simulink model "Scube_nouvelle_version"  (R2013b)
settings: Solver=ode23t  StartTime=0.0  StopTime=100  RelTol=1e-3
libraries: fl_lib x14, nesl_utility x7

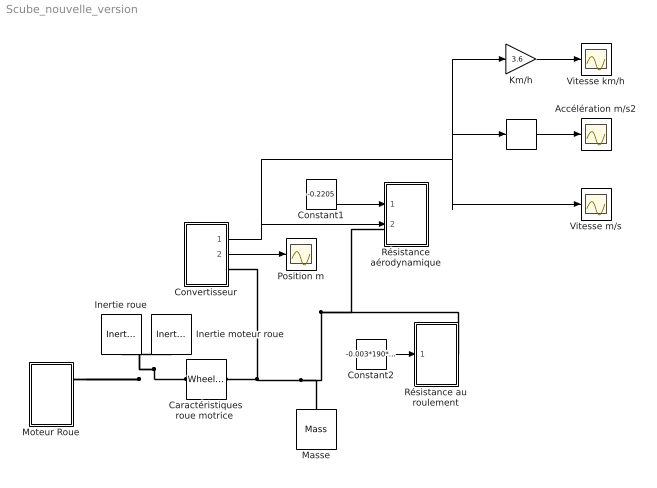
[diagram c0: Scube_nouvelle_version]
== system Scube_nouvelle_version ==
  " " : Derivative
  Accélération m/s2 : Scope
  "Caractéristiques roue motrice " : fl_lib/Mechanical/Mechanisms/Wheel and Axle  R=50 mm  or=1  orient=1  t_Log=off  f_Log=off  LocalVarNames=|t|f  LocalVarDescs=|t|f  LocalVarLogging=[0 0]
  Constant1 : Constant  Value=-0.2205
  Constant2 : Constant  Value=-0.003*190*9.81
  Convertisseur : Subsystem
  Inertie moteur roue : fl_lib/Mechanical/Rotational Elements/Inertia  inertia=0.01 kg*m^2  initial_velocity=0 rad/s  t_Log=off  LocalVarNames=|t  LocalVarDescs=|t  LocalVarLogging=0
  Inertie roue : fl_lib/Mechanical/Rotational Elements/Inertia  inertia=0.01 kg*m^2  initial_velocity=0 rad/s  t_Log=off  LocalVarNames=|t  LocalVarDescs=|t  LocalVarLogging=0
  Km/h : Gain  Gain=3.6
  Masse : fl_lib/Mechanical/Translational Elements/Mass  mass=190 kg  initial_velocity=0 m/s  f_Log=off  LocalVarNames=|f  LocalVarDescs=|f  LocalVarLogging=0
  Moteur Roue : Subsystem
  Position m : Scope
  Résistance au roulement : Subsystem
  Résistance aérodynamique : Subsystem
  Vitesse km/h : Scope
  Vitesse m/s : Scope
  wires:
  Km/h/1 -> Vitesse km/h/1
  " "/1 -> Accélération m/s2/1
  Convertisseur/1(m/s) -> Km/h/1, " "/1, Vitesse m/s/1, Résistance aérodynamique/2(In2)
  Convertisseur/2(m) -> Position m/1
  Constant2/1 -> Résistance au roulement/1(In1)
  Constant1/1 -> Résistance aérodynamique/1(In1)
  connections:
  "Caractéristiques roue motrice "/LConn1 -- Moteur Roue/RConn1 -- Moteur Roue/RConn2 -- Inertie moteur roue/LConn1 -- Inertie roue/LConn1
  Résistance au roulement/RConn1 -- Résistance aérodynamique/LConn1 -- Masse/LConn1 -- Convertisseur/RConn1 -- "Caractéristiques roue motrice "/RConn1

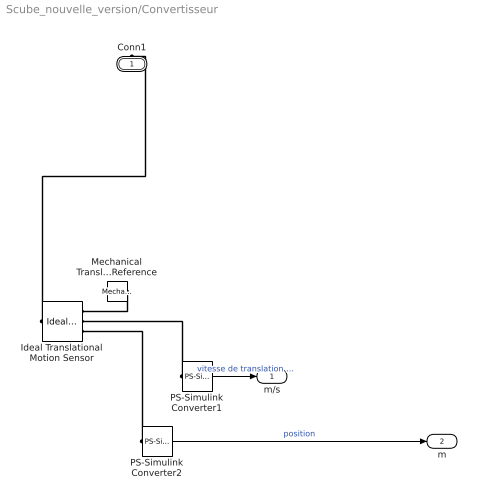
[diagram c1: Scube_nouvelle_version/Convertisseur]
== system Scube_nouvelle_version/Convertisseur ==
  Ideal Translational Motion Sensor : fl_lib/Mechanical/Mechanical Sensors/Ideal Translational Motion Sensor  offset=0 m  v_Log=off  f_Log=off  x_Log=off  LocalVarNames=|v|f|x  LocalVarDescs=|v|f|x  LocalVarLogging=[0 0 0]
  Mechanical Translational Reference : fl_lib/Mechanical/Translational Elements/Mechanical Translational Reference  f_Log=off  LocalVarNames=|f  LocalVarDescs=|f  LocalVarLogging=0
  PS-Simulink Converter1 : nesl_utility/PS-Simulink Converter  PhysicalDomain=network_engine_domain  SubClassName=ps_output  LeftPortType=input  RightPortType=output  PseudoPeriodic=off  Frequencies=[]  Unit=m/s  AffineConversion=off
  PS-Simulink Converter2 : nesl_utility/PS-Simulink Converter  PhysicalDomain=network_engine_domain  SubClassName=ps_output  LeftPortType=input  RightPortType=output  PseudoPeriodic=off  Frequencies=[]  Unit=m  AffineConversion=off
  Conn1 : PMIOPort  Port=1  Side=Right
  m/s : Outport
  m : Outport  Port=2
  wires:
  PS-Simulink Converter1/1 -> m/s/1  "vitesse de translation  de l'axe en m/s"
  PS-Simulink Converter2/1 -> m/1  "position"
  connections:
  PS-Simulink Converter2/LConn1 -- Ideal Translational Motion Sensor/RConn3
  Ideal Translational Motion Sensor/LConn1 -- Conn1/RConn1
  PS-Simulink Converter1/LConn1 -- Ideal Translational Motion Sensor/RConn2
  Mechanical Translational Reference/LConn1 -- Ideal Translational Motion Sensor/RConn1

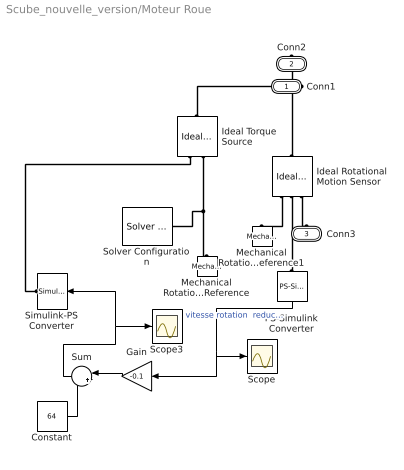
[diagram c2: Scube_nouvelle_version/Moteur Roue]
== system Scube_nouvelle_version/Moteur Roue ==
  Constant : Constant  Value=64
  Gain : Gain  Gain=-0.1
  Ideal Rotational Motion Sensor : fl_lib/Mechanical/Mechanical Sensors/Ideal Rotational Motion Sensor  offset=0 rad  w_Log=off  t_Log=off  phi_Log=off  LocalVarNames=|w|t|phi  LocalVarDescs=|w|t|phi  LocalVarLogging=[0 0 0]
  Ideal Torque Source : fl_lib/Mechanical/Mechanical Sources/Ideal Torque Source  w_Log=off  t_Log=off  LocalVarNames=|w|t  LocalVarDescs=|w|t  LocalVarLogging=[0 0]
  Mechanical Rotational Reference : fl_lib/Mechanical/Rotational Elements/Mechanical Rotational Reference  t_Log=off  LocalVarNames=|t  LocalVarDescs=|t  LocalVarLogging=0
  Mechanical Rotational Reference1 : fl_lib/Mechanical/Rotational Elements/Mechanical Rotational Reference  t_Log=off  LocalVarNames=|t  LocalVarDescs=|t  LocalVarLogging=0
  PS-Simulink Converter : nesl_utility/PS-Simulink Converter  PhysicalDomain=network_engine_domain  SubClassName=ps_output  LeftPortType=input  RightPortType=output  PseudoPeriodic=off  Frequencies=[]  Unit=rpm  AffineConversion=off
  Scope : Scope
  Scope3 : Scope
  Simulink-PS Converter : nesl_utility/Simulink-PS Converter  PhysicalDomain=network_engine_domain  SubClassName=ps_input  LeftPortType=input  RightPortType=output  PseudoPeriodic=off  Frequencies=[]  NoiseDistribution=none  NoiseParameters=[]  Unit=1  AffineConversion=off  InputFiltering=off  SimscapeFilterOrder=1  InputFilterTimeConstant=0.001  UdotUserProvided=1
  Solver Configuration : nesl_utility/Solver Configuration  PhysicalDomain=network_engine_domain  SubClassName=solver  LeftPortType=input  RightPortType=generic  Accelerate=off  Tones=[]  Harmonics=[]  SimulateNoise=off  Profile=off  UseLocalSampling=off  EnableSwitchedLinearOptims=on  FrequencyDomain=off  UseCCode=off  RelTol=0.001  AbsTol=1e-06  MinStep=1e-09  ToWorkspace=off  DoDC=off  ResidualTolerance=1e-9  UseLocalSolver=off  LocalSolverChoice=NE_BACKWARD_EULER_ADVANCER  LocalSolverSampleTime=.001  DoFixedCost=off  MaxNonlinIter=3  MaxModeIter=2  LinearAlgebra=Sparse  DelaysMemoryBudget=1024
  Sum : Sum  Inputs=|++
  Conn1 : PMIOPort  Port=1  Side=Right
  Conn2 : PMIOPort  Port=2  Side=Right
  Conn3 : PMIOPort  Port=3  Side=Left
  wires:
  PS-Simulink Converter/1 -> Gain/1, Scope/1  "vitesse rotation  reducteur en tr/min"
  Sum/1 -> Simulink-PS Converter/1, Scope3/1
  Constant/1 -> Sum/2
  Gain/1 -> Sum/1
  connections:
  Ideal Rotational Motion Sensor/RConn3 -- Conn3/RConn1
  Ideal Torque Source/LConn1 -- Conn1/RConn1
  Ideal Torque Source/RConn2 -- Mechanical Rotational Reference/LConn1 -- Solver Configuration/RConn1
  Ideal Rotational Motion Sensor/RConn2 -- PS-Simulink Converter/LConn1
  Ideal Rotational Motion Sensor/LConn1 -- Conn2/RConn1
  Ideal Torque Source/RConn1 -- Simulink-PS Converter/RConn1
  Ideal Rotational Motion Sensor/RConn1 -- Mechanical Rotational Reference1/LConn1

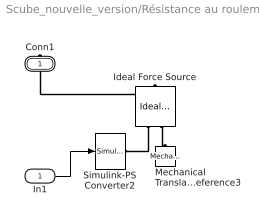
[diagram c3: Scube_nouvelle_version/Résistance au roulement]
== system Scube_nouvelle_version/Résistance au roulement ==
  In1 : Inport
  Ideal Force Source : fl_lib/Mechanical/Mechanical Sources/Ideal Force Source  v_Log=off  f_Log=off  LocalVarNames=|v|f  LocalVarDescs=|v|f  LocalVarLogging=[0 0]
  Mechanical Translational Reference3 : fl_lib/Mechanical/Translational Elements/Mechanical Translational Reference  f_Log=off  LocalVarNames=|f  LocalVarDescs=|f  LocalVarLogging=0
  Simulink-PS Converter2 : nesl_utility/Simulink-PS Converter  PhysicalDomain=network_engine_domain  SubClassName=ps_input  LeftPortType=input  RightPortType=output  PseudoPeriodic=off  Frequencies=[]  NoiseDistribution=none  NoiseParameters=[]  Unit=1  AffineConversion=off  InputFiltering=off  SimscapeFilterOrder=1  InputFilterTimeConstant=0.001  UdotUserProvided=1
  Conn1 : PMIOPort  Port=1  Side=Right
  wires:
  In1/1 -> Simulink-PS Converter2/1
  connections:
  Ideal Force Source/LConn1 -- Conn1/RConn1
  Ideal Force Source/RConn1 -- Simulink-PS Converter2/RConn1
  Ideal Force Source/RConn2 -- Mechanical Translational Reference3/LConn1

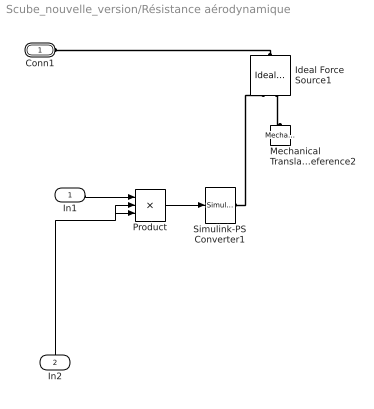
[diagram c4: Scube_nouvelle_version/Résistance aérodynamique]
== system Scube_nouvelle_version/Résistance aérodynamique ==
  In1 : Inport
  In2 : Inport  Port=2
  Ideal Force Source1 : fl_lib/Mechanical/Mechanical Sources/Ideal Force Source  v_Log=off  f_Log=off  LocalVarNames=|v|f  LocalVarDescs=|v|f  LocalVarLogging=[0 0]
  Mechanical Translational Reference2 : fl_lib/Mechanical/Translational Elements/Mechanical Translational Reference  f_Log=off  LocalVarNames=|f  LocalVarDescs=|f  LocalVarLogging=0
  Product : Product  Inputs=3
  Simulink-PS Converter1 : nesl_utility/Simulink-PS Converter  PhysicalDomain=network_engine_domain  SubClassName=ps_input  LeftPortType=input  RightPortType=output  PseudoPeriodic=off  Frequencies=[]  NoiseDistribution=none  NoiseParameters=[]  Unit=1  AffineConversion=off  InputFiltering=off  SimscapeFilterOrder=1  InputFilterTimeConstant=0.001  UdotUserProvided=1
  Conn1 : PMIOPort  Port=1  Side=Left
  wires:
  Product/1 -> Simulink-PS Converter1/1
  In1/1 -> Product/1
  In2/1 -> Product/2, Product/3
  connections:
  Ideal Force Source1/RConn2 -- Mechanical Translational Reference2/LConn1
  Simulink-PS Converter1/RConn1 -- Ideal Force Source1/RConn1
  Ideal Force Source1/LConn1 -- Conn1/RConn1
